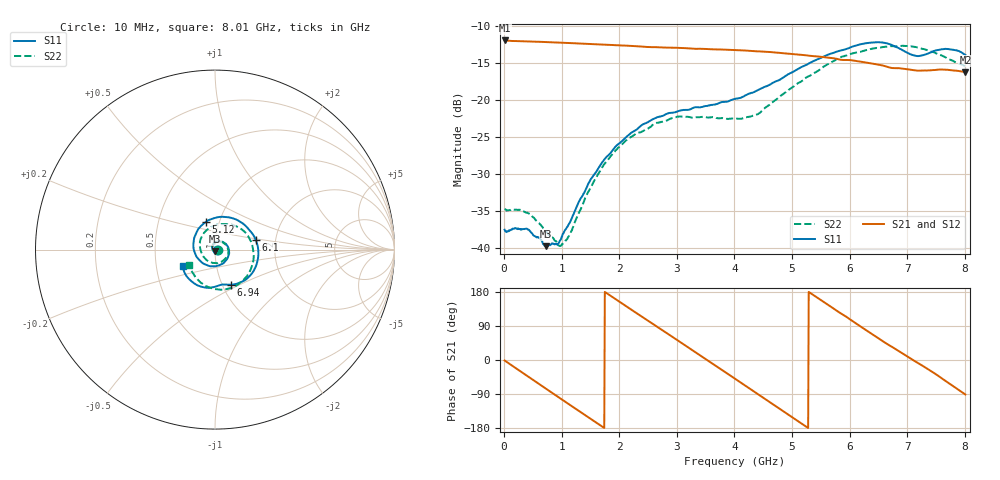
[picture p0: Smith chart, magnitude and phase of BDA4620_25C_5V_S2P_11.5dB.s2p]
!Agilent Technologies,E5071B,MY42404982,A.09.10
!Date: Wed May 06 09:00:34 2026
!Data & Calibration Information:
!Freq	S11:SOLT2(ON)	S21:SOLT2(ON)	S12:SOLT2(ON)	S22:SOLT2(ON)
# Hz S RI R 50
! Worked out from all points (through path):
!   801 points, 10 MHz to 8.01 GHz, reference 50 ohm
!   highest |S21| = -11.94 dB at 10 MHz (marker M1); lowest = -16.2 dB at 8.01 GHz (marker M2)
!   group delay of S21, straight-line fit = 281 ps
!   lowest |S11| = -39.8 dB at 720 MHz (marker M3), VSWR 1.02, Z = 50 - j1.02 ohm
!   |S11| at or under -10 dB: start of sweep to end of sweep
!   |S22| runs from -39.8 to -12.7 dB; largest |S21 - S12| = 0.001
!   S11 on the Smith chart (normalised r, x): 10 MHz: 1.03, -0.00; 5.12 GHz: 0.87, +0.28; 6.1 GHz: 1.57, +0.19; 6.94 GHz: 1.10, -0.45; 8.01 GHz: 0.69, -0.13
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1e7  0.0132 -0.000848  0.253 -0.00541  0.2533 -0.00558  0.0182 -0.00108
4e8  0.0106 -0.00823  0.1858 -0.1663  0.186 -0.1667  0.0143 -0.0096
7.2e8  0.000448 -0.0102  0.0643 -0.2384  0.0643 -0.2387  0.00351 -0.0127
1e9  -0.011 -0.00426  -0.0579 -0.2374  -0.0581 -0.2377  -0.00817 -0.00636
1.35e9  -0.0164 0.0148  -0.1836 -0.1562  -0.1837 -0.1563  -0.0146 0.012
1.6e9  -0.0091 0.0313  -0.2305 -0.0613  -0.2307 -0.0615  -0.00961 0.0284
1.92e9  0.0136 0.0455  -0.2243 0.0714  -0.2245 0.0717  0.0104 0.0434
2.32e9  0.0515 0.0379  -0.121 0.1967  -0.1214 0.197  0.045 0.0393
2.68e9  0.0767 0.00476  0.0178 0.2269  0.018 0.2271  0.0686 0.0148
3.39e9  0.0367 -0.0812  0.2158 0.0531  0.2161 0.0528  0.0466 -0.0606
4.01e9  -0.0681 -0.0754  0.1418 -0.1653  0.1418 -0.1657  -0.0426 -0.0615
4.53e9  -0.1208 0.0224  -0.0466 -0.2074  -0.0468 -0.2078  -0.0858 0.0212
5.12e9  -0.0488 0.1564  -0.1941 -0.0591  -0.1944 -0.0588  -0.0121 0.1304
5.35e9  0.0176 0.1808  -0.1973 0.0223  -0.1975 0.0224  0.045 0.142
5.68e9  0.1252 0.1641  -0.1476 0.1238  -0.1476 0.1243  0.1305 0.1235
6.1e9  0.2264 0.0562  -0.0244 0.1825  -0.0243 0.1828  0.2074 0.0247
6.39e9  0.2377 -0.0599  0.0654 0.1638  0.0654 0.1639  0.2137 -0.0621
6.68e9  0.1756 -0.1638  0.1284 0.106  0.1288 0.1062  0.1786 -0.1461
6.94e9  0.0902 -0.1952  0.1572 0.0424  0.1576 0.0424  0.1176 -0.201
7.19e9  0.0362 -0.1948  0.1563 -0.0228  0.1568 -0.0228  0.0368 -0.2236
7.59e9  -0.0737 -0.2074  0.1092 -0.1181  0.1094 -0.1184  -0.0777 -0.1849
8.01e9  -0.1793 -0.0927  -0.00282 -0.1542  -0.00275 -0.1546  -0.1447 -0.0862
